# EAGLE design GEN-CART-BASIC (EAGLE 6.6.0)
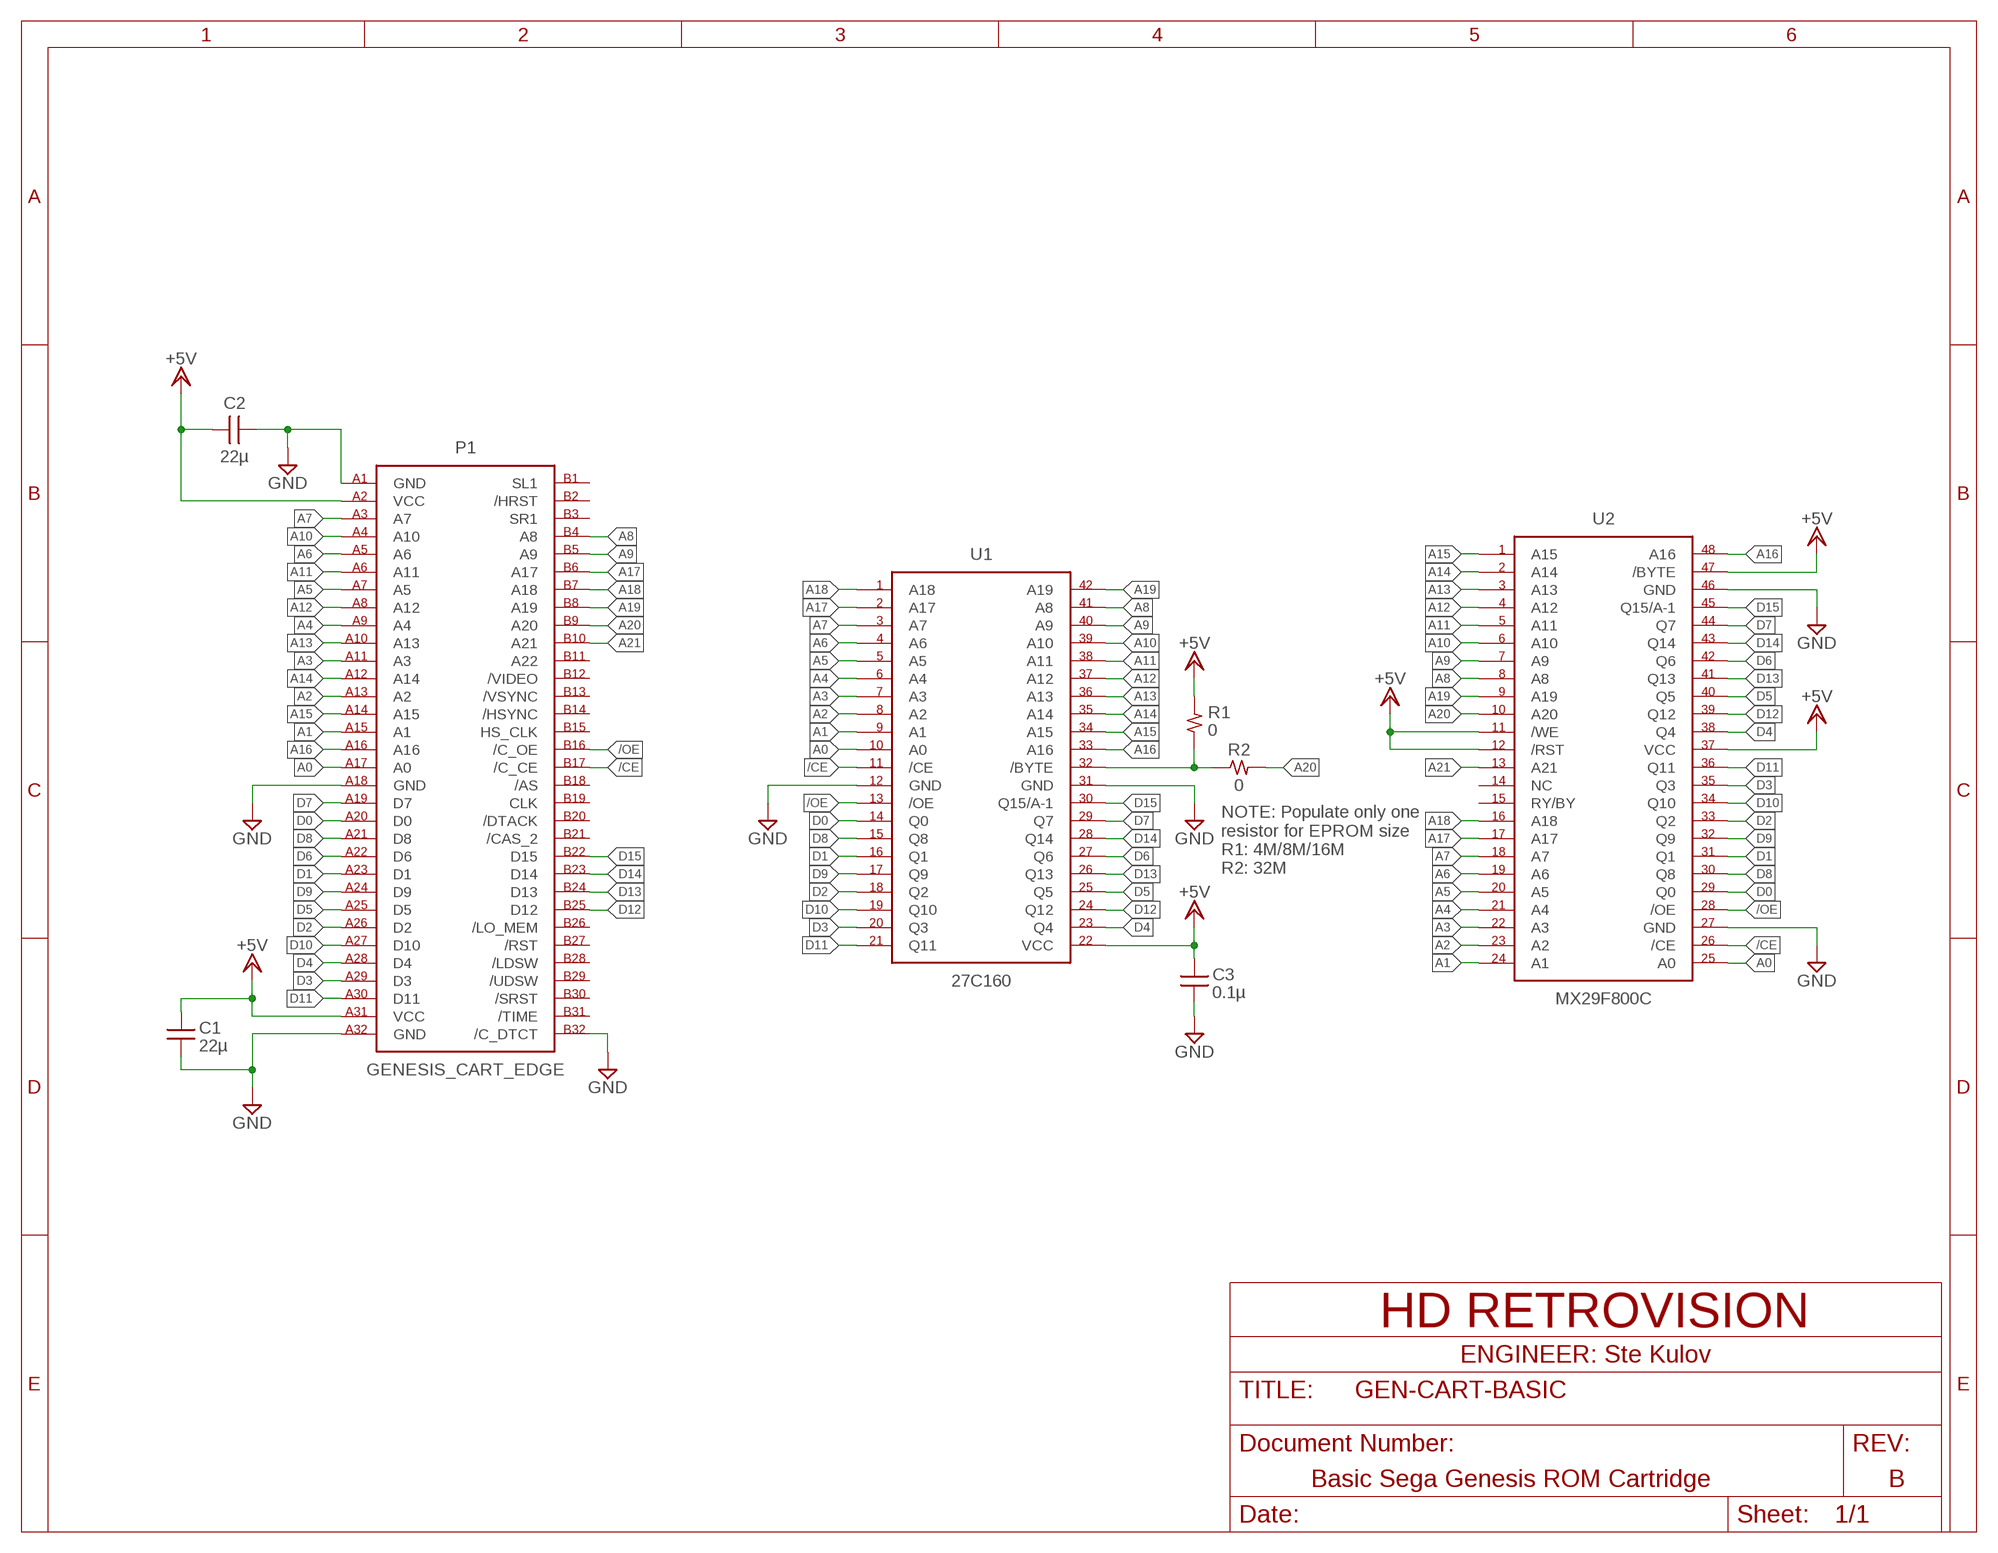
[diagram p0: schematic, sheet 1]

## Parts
C1  22µ  CAP_SMD1210  [CAP_SMD1210]
C2  22µ  CAP_SMD_HORIZONTAL1210  [CAP_SMD1210]
C3  0.1µ  CAP_SMD0603  [CAP_SMD0603]
P1  GENESIS_CART_EDGE  [GENESIS_CART_EDGE]
R1  0  RES_SMD0603  [RES_SMD0603]
R2  0  RES_SMD_HORIZONTAL0603  [RES_SMD0603]
U1  27C160  [DIP_600MIL_42]
U2  MX29F800C  [TSOP48]

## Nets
/CE: P1.B17(/C_CE) U1.P$11(/CE) U2.P$26(/CE)
/OE: P1.B16(/C_OE) U1.P$13(/OE) U2.P$28(/OE)
A0: P1.A17(A0) U1.P$10(A0) U2.P$25(A0)
A1: P1.A15(A1) U1.P$9(A1) U2.P$24(A1)
A2: P1.A13(A2) U1.P$8(A2) U2.P$23(A2)
A3: P1.A11(A3) U1.P$7(A3) U2.P$22(A3)
A4: P1.A9(A4) U1.P$6(A4) U2.P$21(A4)
A5: P1.A7(A5) U1.P$5(A5) U2.P$20(A5)
A6: P1.A5(A6) U1.P$4(A6) U2.P$19(A6)
A7: P1.A3(A7) U1.P$3(A7) U2.P$18(A7)
A8: P1.B4(A8) U1.P$41(A8) U2.P$8(A8)
A9: P1.B5(A9) U1.P$40(A9) U2.P$7(A9)
A10: P1.A4(A10) U1.P$39(A10) U2.P$6(A10)
A11: P1.A6(A11) U1.P$38(A11) U2.P$5(A11)
A12: P1.A8(A12) U1.P$37(A12) U2.P$4(A12)
A13: P1.A10(A13) U1.P$36(A13) U2.P$3(A13)
A14: P1.A12(A14) U1.P$35(A14) U2.P$2(A14)
A15: P1.A14(A15) U1.P$34(A15) U2.P$1(A15)
A16: P1.A16 U1.P$33(A16) U2.P$48(A16)
A17: P1.B6(A17) U1.P$2(A17) U2.P$17(A17)
A18: P1.B7(A18) U1.P$1(A18) U2.P$16(A18)
A19: P1.B8(A19) U1.P$42(A19) U2.P$9(A19)
A20: P1.B9(A20) R2.P$2 U2.P$10(A20)
A21: P1.B10(A21) U2.P$13(A21)
D0: P1.A20(D0) U1.P$14(Q0) U2.P$29(Q0)
D1: P1.A23(D1) U1.P$16(Q1) U2.P$31(Q1)
D2: P1.A26(D2) U1.P$18(Q2) U2.P$33(Q2)
D3: P1.A29(D3) U1.P$20(Q3) U2.P$35(Q3)
D4: P1.A28(D4) U1.P$23(Q4) U2.P$38(Q4)
D5: P1.A25(D5) U1.P$25(Q5) U2.P$40(Q5)
D6: P1.A22(D6) U1.P$27(Q6) U2.P$42(Q6)
D7: P1.A19(D7) U1.P$29(Q7) U2.P$44(Q7)
D8: P1.A21(D8) U1.P$15(Q8) U2.P$30(Q8)
D9: P1.A24(D9) U1.P$17(Q9) U2.P$32(Q9)
D10: P1.A27(D10) U1.P$19(Q10) U2.P$34(Q10)
D11: P1.A30(D11) U1.P$21(Q11) U2.P$36(Q11)
D12: P1.B25(D12) U1.P$24(Q12) U2.P$39(Q12)
D13: P1.B24(D13) U1.P$26(Q13) U2.P$41(Q13)
D14: P1.B23(D14) U1.P$28(Q14) U2.P$43(Q14)
D15: P1.B22(D15) U1.P$30(Q15/A-1) U2.P$45(Q15/A-1)
GND: C1.P$1 C2.P$1 C3.P$1 P1.A1(GND) P1.A18(GND) P1.A32(GND) P1.B32(/C_DTCT) U1.P$12(GND) U1.P$31(GND) U2.P$27(GND) U2.P$46(GND)
N$5: R1.P$1 R2.P$1 U1.P$32(/BYTE)
V+: C1.P$2 C2.P$2 C3.P$2 P1.A2(VCC) P1.A31(VCC) R1.P$2 U1.P$22(VCC) U2.P$11(/WE) U2.P$12(/RST) U2.P$37(VCC) U2.P$47(/BYTE) ; supply symbol labelled +5V
Unconnected: P1.B1(SL1) P1.B2(/HRST) P1.B3(SR1) P1.B11(A22) P1.B12(/VIDEO) P1.B13(/VSYNC) P1.B14(/HSYNC) P1.B15(HS_CLK) P1.B18(/AS) P1.B19(CLK) P1.B20(/DTACK) P1.B21(/CAS_2) P1.B26(/LO_MEM) P1.B27(/RST) P1.B28(/LDSW) P1.B29(/UDSW) P1.B30(/SRST) P1.B31(/TIME) U2.P$14(NC) U2.P$15(RY/BY)

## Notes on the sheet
- NOTE: Populate only one
  resistor for EPROM size
  R1: 4M/8M/16M
  R2: 32M
- HD RETROVISION
- ENGINEER: Ste Kulov
- Basic Sega Genesis ROM Cartridge | B

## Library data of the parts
C1 C3 = hdretrovision:CAP_SMD
C2 = hdretrovision:CAP_SMD_HORIZONTAL
P1 = hdretrovision:GENESIS_CART_EDGE
R1 = hdretrovision:RES_SMD
R2 = hdretrovision:RES_SMD_HORIZONTAL
U1 = hdretrovision:27C160
U2 = hdretrovision:MX29F800C

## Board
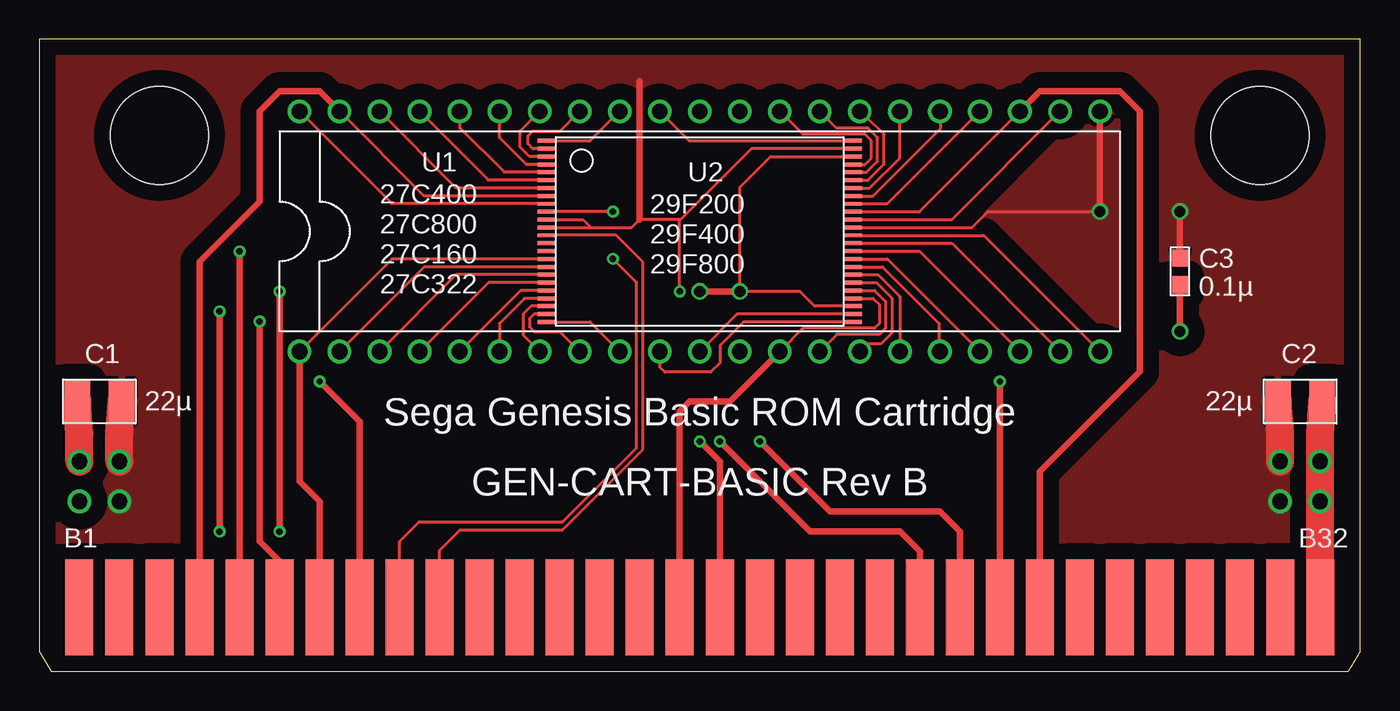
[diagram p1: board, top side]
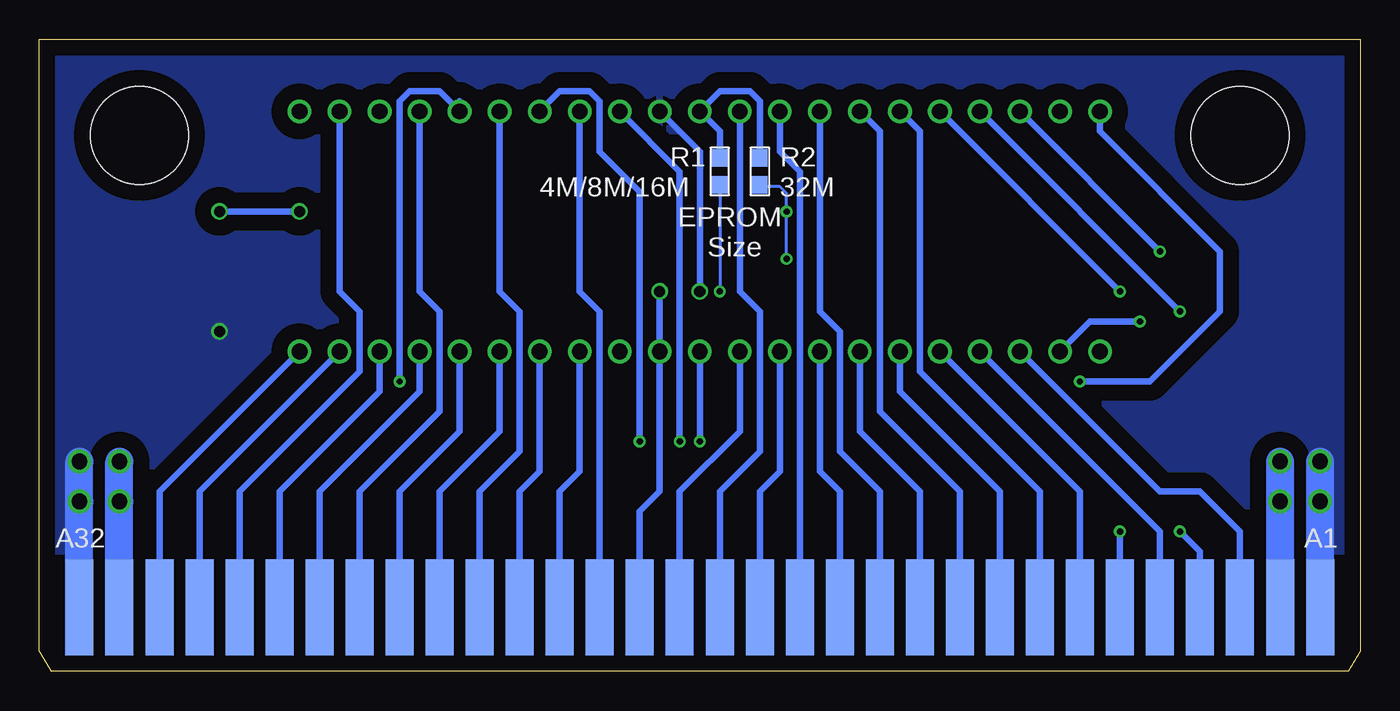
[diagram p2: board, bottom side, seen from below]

Size 83.82 x 40.13 mm. Coordinates in mm from the lower left corner, seen from the top.
Outline: 0.76,0 83.06,0 83.82,1.27 83.82,40.13 0,40.13 0,1.27 0.76,0
Copper layers (1*16): Top 0.0356mm / dielectric 1.5011mm / Bottom 0.0356mm
Design rules "LaenPCBOrder": minimum track width 6mil, minimum drill 13mil, track to track 6mil, track to pad 6mil, pad to pad 6mil, via to via 6mil, smd to smd 6mil, copper to edge 15mil, drill to drill 6mil, minimum pad ring 7mil, minimum via ring 7mil, stop-mask expansion 4mil, vias tented up to drill 0mil, thermal gap 10mil
Holes 6.22 mm at 7.62,34.04 77.47,34.04

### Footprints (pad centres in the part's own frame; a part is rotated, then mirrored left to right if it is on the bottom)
CAP_SMD1210 = smd 1.6 x 2.7: P$1 -1.4,0; P$2 1.4,0
CAP_SMD0603 = smd 1.1 x 1: P$1 -0.85,0; P$2 0.85,0
GENESIS_CART_EDGE = smd 1.778 x 6.096 bottom: A1 -38.1,0; A2 -35.56,0; A3 -33.02,0; A4 -30.48,0; A5 -27.94,0; A6 -25.4,0; A7 -22.86,0; A8 -20.32,0; A9 -17.78,0; A10 -15.24,0; A11 -12.7,0; A12 -10.16,0; A13 -7.62,0; A14 -5.08,0; A15 -2.54,0; A16 0,0; A17 2.54,0; A18 5.08,0; A19 7.62,0; A20 10.16,0; A21 12.7,0; A22 15.24,0; A23 17.78,0; A24 20.32,0; A25 22.86,0; A26 25.4,0; A27 27.94,0; A28 30.48,0; A29 33.02,0; A30 35.56,0; A31 38.1,0; A32 40.64,0 | smd 1.778 x 6.096: B1 -38.1,0; B2 -35.56,0; B3 -33.02,0; B4 -30.48,0; B5 -27.94,0; B6 -25.4,0; B7 -22.86,0; B8 -20.32,0; B9 -17.78,0; B10 -15.24,0; B11 -12.7,0; B12 -10.16,0; B13 -7.62,0; B14 -5.08,0; B15 -2.54,0; B16 0,0; B17 2.54,0; B18 5.08,0; B19 7.62,0; B20 10.16,0; B21 12.7,0; B22 15.24,0; B23 17.78,0; B24 20.32,0; B25 22.86,0; B26 25.4,0; B27 27.94,0; B28 30.48,0; B29 33.02,0; B30 35.56,0; B31 38.1,0; B32 40.64,0
RES_SMD0603 = smd 1.1 x 1: P$1 -0.85,0; P$2 0.85,0
DIP_600MIL_42 = drill 1: P$1 -25.4,-7.62; P$2 -22.86,-7.62; P$3 -20.32,-7.62; P$4 -17.78,-7.62; P$5 -15.24,-7.62; P$6 -12.7,-7.62; P$7 -10.16,-7.62; P$8 -7.62,-7.62; P$9 -5.08,-7.62; P$10 -2.54,-7.62; P$11 0,-7.62; P$12 2.54,-7.62; P$13 5.08,-7.62; P$14 7.62,-7.62; P$15 10.16,-7.62; P$16 12.7,-7.62; P$17 15.24,-7.62; P$18 17.78,-7.62; P$19 20.32,-7.62; P$20 22.86,-7.62; P$21 25.4,-7.62; P$22 25.4,7.62; P$23 22.86,7.62; P$24 20.32,7.62; P$25 17.78,7.62; P$26 15.24,7.62; P$27 12.7,7.62; P$28 10.16,7.62; P$29 7.62,7.62; P$30 5.08,7.62; P$31 2.54,7.62; P$32 0,7.62; P$33 -2.54,7.62; P$34 -5.08,7.62; P$35 -7.62,7.62; P$36 -10.16,7.62; P$37 -12.7,7.62; P$38 -15.24,7.62; P$39 -17.78,7.62; P$40 -20.32,7.62; P$41 -22.86,7.62; P$42 -25.4,7.62
TSOP48 = smd 1.1 x 0.25: P$1 -9.75,5.75; P$2 -9.75,5.25; P$3 -9.75,4.75; P$4 -9.75,4.25; P$5 -9.75,3.75; P$6 -9.75,3.25; P$7 -9.75,2.75; P$8 -9.75,2.25; P$9 -9.75,1.75; P$10 -9.75,1.25; P$11 -9.75,0.75; P$12 -9.75,0.25; P$13 -9.75,-0.25; P$14 -9.75,-0.75; P$15 -9.75,-1.25; P$16 -9.75,-1.75; P$17 -9.75,-2.25; P$18 -9.75,-2.75; P$19 -9.75,-3.25; P$20 -9.75,-3.75; P$21 -9.75,-4.25; P$22 -9.75,-4.75; P$23 -9.75,-5.25; P$24 -9.75,-5.75; P$25 9.75,-5.75; P$26 9.75,-5.25; P$27 9.75,-4.75; P$28 9.75,-4.25; P$29 9.75,-3.75; P$30 9.75,-3.25; P$31 9.75,-2.75; P$32 9.75,-2.25; P$33 9.75,-1.75; P$34 9.75,-1.25; P$35 9.75,-0.75; P$36 9.75,-0.25; P$37 9.75,0.25; P$38 9.75,0.75; P$39 9.75,1.25; P$40 9.75,1.75; P$41 9.75,2.25; P$42 9.75,2.75; P$43 9.75,3.25; P$44 9.75,3.75; P$45 9.75,4.25; P$46 9.75,4.75; P$47 9.75,5.25; P$48 9.75,5.75

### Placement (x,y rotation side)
C1  3.81,17.14 0 top
C2  80.01,17.14 180 top
C3  72.39,25.4 90 top
P1  40.64,4.06 0 top
R1  40.64,31.75 270 bottom
R2  38.1,31.75 270 bottom
U1  41.91,27.94 0 top
U2  41.91,27.94 0 top

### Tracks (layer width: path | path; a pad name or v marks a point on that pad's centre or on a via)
/CE  (via drill 0.4)
  Top 0.2: U2.P$26 44.28,22.69 U1.P$11
  Top 0.406: P1.B17 43.18,13.34 v41.91,14.61
  Bottom 0.406: v41.91,14.61 U1.P$11
/OE
  Top 0.2: U2.P$28 52.91,23.69 53.3,23.3 53.3,22.1 53,21.8 48.47,21.8 U1.P$13
  Top 0.406: P1.B16 40.64,16.51 41.27,17.14 43.81,17.14 U1.P$13
A0
  Top 0.2: U2.P$25 44.69,22.19 43.2,20.7 43.2,19.6 42.6,19 39.7,19 39.4,19.3 39.4,20.29 U1.P$10
  Bottom 0.406: P1.A17 43.18,11.43 39.37,15.24 U1.P$10
A1
  Top 0.2: U2.P$24 34.96,22.19 U1.P$9
  Bottom 0.406: P1.A15 38.1,11.43 36.83,12.7 U1.P$9
A2
  Top 0.2: U2.P$23 31.39,22.69 31.1,22.4 31.1,21.9 31.4,21.6 33.01,21.6 U1.P$8
  Bottom 0.406: P1.A13 33.02,11.43 34.29,12.7 U1.P$8
A3
  Top 0.2: U2.P$22 31.19,23.19 30.7,22.7 30.7,21.37 U1.P$7
  Bottom 0.406: P1.A11 27.94,11.43 31.75,15.24 U1.P$7
A4
  Top 0.2: U2.P$21 30.79,23.69 29.2,22.1 U1.P$6
  Bottom 0.406: P1.A9 22.86,11.43 29.21,17.78 U1.P$6
A5
  Top 0.2: U2.P$20 30.54,24.19 U1.P$5
  Bottom 0.406: P1.A7 17.78,11.43 U1.P$5
A6
  Top 0.2: U2.P$19 28.5,24.69 U1.P$4
  Bottom 0.406: P1.A5 12.7,8.89 U1.P$4
A7
  Top 0.2: U2.P$18 26.46,25.19 U1.P$3
  Bottom 0.406: P1.A3 7.62,8.89 10.16,11.43 12.7,11.43 U1.P$3
A8
  Top 0.2: U2.P$8 24.42,30.19 U1.P$41
  Top 0.406: P1.B4 10.16,26.04 13.97,29.84 13.97,35.56 15.24,36.83 17.78,36.83 U1.P$41
A9  (via drill 0.4)
  Top 0.2: U2.P$7 26.46,30.69 U1.P$40
  Top 0.406: P1.B5 v12.7,26.67
  Bottom 0.406: v12.7,26.67 U1.P$40
A10  (via drill 0.4)
  Top 0.2: U2.P$6 28.5,31.19 U1.P$39
  Top 0.406: v11.43,8.89 v11.43,22.86
  Bottom 0.406: P1.A4 10.16,7.62 v11.43,8.89 | v11.43,22.86 U1.P$39
A11  (via drill 0.4)
  Top 0.2: U2.P$5 29.51,31.69 26.7,34.5 26.7,35.53 U1.P$38
  Top 0.406: v15.24,8.89 v15.24,24.13
  Bottom 0.406: v15.24,24.13 U1.P$38 | P1.A6 v15.24,8.89
A12
  Top 0.2: U2.P$4 30.91,32.19 29.2,33.9 U1.P$37
  Bottom 0.406: P1.A8 20.32,11.43 27.94,19.05 27.94,34.29 U1.P$37
A13
  Top 0.2: U2.P$3 31.11,32.69 30.5,33.3 30.5,34.31 U1.P$36
  Bottom 0.406: P1.A10 25.4,11.43 30.48,16.51 30.48,34.29 U1.P$36
A14
  Top 0.2: U2.P$2 31.31,33.19 31,33.5 31,34 31.3,34.3 33.03,34.3 U1.P$35
  Bottom 0.406: P1.A12 30.48,11.43 33.02,13.97 33.02,21.59 34.29,22.86 U1.P$35
A15
  Top 0.2: U2.P$1 34.96,33.69 U1.P$34
  Bottom 0.406: P1.A14 35.56,31.75 36.83,33.02 U1.P$34
A16
  Top 0.2: U1.P$33 41.23,33.7 42.5,33.7 42.51,33.69 U2.P$48
  Bottom 0.406: P1.A16 40.64,11.43 38.1,13.97 38.1,22.86 39.37,24.13 U1.P$33
A17  (via drill 0.4)
  Top 0.2: U2.P$17 24.42,25.69 U1.P$2
  Top 0.406: P1.B6 15.24,6.99 13.97,8.26 v13.97,22.23
  Bottom 0.406: v13.97,22.23 17.14,22.23 U1.P$2
A18
  Top 0.2: U2.P$16 22.38,26.19 U1.P$1
  Top 0.406: P1.B7 17.78,10.79 16.51,12.06 U1.P$1
A19  (via drill 0.4)
  Top 0.2: U2.P$9 22.38,29.69 U1.P$42
  Top 0.406: P1.B8 20.32,15.88 v17.78,18.41
  Bottom 0.406: v17.78,18.41 13.34,18.41 8.89,22.86 8.89,26.67 16.51,34.29 U1.P$42
A20  (via drill 0.4)
  Top 0.2: P1.B9 22.86,8.26 24.1,9.5 33.2,9.5 37.9,14.2 37.9,24.7 v36.4,26.2 | v36.4,29.2 U2.P$10
  Bottom 0.2: v36.4,26.2 v36.4,29.2 36.4,30.37 36.83,30.8 38,30.8 R2.P$2
A21
  Top 0.2: P1.B10 25.4,7.7 26.7,9 33.2,9 38.3,14.1 38.3,26 36.6,27.7 U2.P$13
D0
  Top 0.2: U2.P$29 53.01,24.19 53.7,23.5 53.7,21.8 53.3,21.4 50.61,21.4 U1.P$14
  Bottom 0.406: P1.A20 50.8,11.43 49.53,12.7 U1.P$14
D1
  Top 0.2: U2.P$31 53.21,25.19 54.6,23.8 U1.P$16
  Bottom 0.406: P1.A23 58.42,11.43 54.61,15.24 U1.P$16
D2
  Top 0.2: U2.P$33 53.82,26.19 U1.P$18
  Bottom 0.406: P1.A26 66.04,11.43 59.69,17.78 U1.P$18
D3
  Top 0.2: U2.P$35 57.9,27.19 U1.P$20
  Bottom 0.406: P1.A29 73.66,11.43 U1.P$20
D4
  Top 0.2: U2.P$38 57.9,28.69 U1.P$23
  Bottom 0.406: P1.A28 71.12,11.43 63.5,19.05 63.5,22.86 64.77,24.13 U1.P$23
D5
  Top 0.2: U2.P$40 53.82,29.69 U1.P$25
  Bottom 0.406: P1.A25 63.5,11.43 58.42,16.51 58.42,22.86 59.69,24.13 U1.P$25
D6
  Top 0.2: U2.P$42 52.69,30.69 54.6,32.6 U1.P$27
  Bottom 0.406: P1.A22 55.88,11.43 53.34,13.97 53.34,22.86 54.61,24.13 U1.P$27
D7
  Top 0.2: U2.P$44 52.49,31.69 53.2,32.4 53.2,33.9 52.6,34.5 50.59,34.5 U1.P$29
  Bottom 0.406: P1.A19 48.26,22.86 49.53,24.13 U1.P$29
D8
  Top 0.2: U2.P$30 53.11,24.69 54.1,23.7 54.1,21.5 53.4,20.8 52.55,20.8 U1.P$15
  Bottom 0.406: P1.A21 53.34,11.43 52.07,12.7 U1.P$15
D9
  Top 0.2: U2.P$32 53.51,25.69 57.1,22.1 57.1,20.37 U1.P$17
  Bottom 0.406: P1.A24 60.96,11.43 57.15,15.24 U1.P$17
D10
  Top 0.2: U2.P$34 55.86,26.69 U1.P$19
  Bottom 0.406: P1.A27 68.58,11.43 62.23,17.78 U1.P$19
D11
  Top 0.2: U2.P$36 59.94,27.69 U1.P$21
  Bottom 0.406: P1.A30 76.2,11.43 U1.P$21
D12
  Top 0.2: U2.P$39 55.86,29.19 U1.P$24
  Top 0.406: P1.B25 63.5,12.7 69.85,19.05 69.85,35.56 68.58,36.83 63.5,36.83 U1.P$24
D13  (via drill 0.4)
  Top 0.2: U2.P$41 52.89,30.19 57.2,34.5 57.2,35.51 U1.P$26
  Top 0.406: P1.B24 v60.96,18.41
  Bottom 0.406: v60.96,18.41 60.96,36.2 60.33,36.83 58.42,36.83 U1.P$26 57.15,36.2
D14  (via drill 0.4)
  Top 0.2: U2.P$43 52.59,31.19 53.6,32.2 53.6,34.1 52.5,35.2 52.43,35.2 U1.P$28
  Top 0.406: P1.B23 58.42,8.89 57.15,10.16 50.16,10.16 v45.72,14.61
  Bottom 0.406: v45.72,14.61 45.72,30.48 48.26,33.02 48.26,36.2 48.9,36.83 50.8,36.83 U1.P$28
D15  (via drill 0.4)
  Top 0.2: U2.P$45 52.39,32.19 52.8,32.6 52.8,33.7 52.4,34.1 48.45,34.1 U1.P$30
  Top 0.406: P1.B22 55.88,7.62 54.61,8.89 48.9,8.89 v43.18,14.61
  Bottom 0.406: v43.18,14.61 43.18,31.75 U1.P$30
GND  (via drill 0.7, 1)
  Top 0.2: U2.P$46 46.4,32.7 44.45,30.75 v44.45,24.13 48.26,24.13 49.2,23.19 U2.P$27
  Top 0.406: C3.P$1 v72.39,21.59 | v41.91,24.13 v44.45,24.13
  Top 1.778: v2.54,13.34 2.54,15.11 C1.P$1 | C2.P$1 81.28,15.11 v81.28,13.34 v81.28,10.79 P1.B32
  Bottom 0.406: P1.A18 45.72,10.16 44.45,11.43 U1.P$12 v44.45,24.13 | U1.P$31 41.91,33.02 v41.91,24.13
  Bottom 1.778: P1.A1 v2.54,10.79 v2.54,13.34 | P1.B32 v81.28,10.79 v81.28,13.34
  pour Bottom (isolate 1.016): 0,7.62 0,40.13 83.82,40.13 83.82,7.62 55.88,7.62 55.88,34.29 27.94,34.29 27.94,7.62
N$5
  Bottom 0.406: R2.P$1 38.1,36.2 38.73,36.83 40.64,36.83 U1.P$32 40.64,34.29 R1.P$1
V+  (via drill 0.4, 0.7, 1)
  Top 0.2: U2.P$12 35,28.19 | 35,28.19 37.59,28.19 38.1,28.7 40.7,28.7 | U2.P$11 34.5,28.69 35,28.19 | U2.P$37 59.19,28.19 60.2,29.2 v67.3,29.2 v67.31,29.21 | U2.P$47 45.19,33.19 40.7,28.7 | v40.64,24.13 40.64,28.64 40.7,28.7
  Top 0.406: U1.P$22 v67.31,29.21 | v72.39,29.21 C3.P$2 | 38.1,28.7 38.1,37.47
  Top 1.778: v5.08,13.34 5.08,15.11 C1.P$2 | v78.74,13.34 78.74,15.11 C2.P$2
  Bottom 0.2: R1.P$2 v40.64,24.13
  Bottom 0.406: v67.31,29.21 v72.39,29.21
  Bottom 1.778: P1.A2 v5.08,10.79 v5.08,13.34 | P1.A31 v78.74,10.79 v78.74,13.34
  pour Top (isolate 1.016): 0,7.62 0,40.13 83.82,40.13 83.82,7.62 55.88,7.62 55.88,34.29 27.94,34.29 27.94,7.62

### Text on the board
tPlace: U1 | U2 | 29F200 / 29F400 / 29F800 | 27C400 / 27C800 / 27C160 / 27C322 | Sega Genesis Basic ROM Cartridge | GEN-CART-BASIC Rev B | B1 | B32
bPlace: 32M | 4M/8M/16M | EPROM | Size | A1 | A32
Reference: Card Edge Detail | 0.063" | 30° | 0.040" | General Fabrication Notes: / / 1.) Board Thickness = 0.063" (1.6mm) / / 2.) Number of Layers = 2 / / 3.) Copper Weight (per layer) = 1oz / / 4.) Gold fingers required on bottom edge / / 5.) Bevel fingered edge as per drawing => / / 6.) Dimension Tolerance = ±0.005" / / 7.) Angle Tolerance = ±2° | 0.017"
